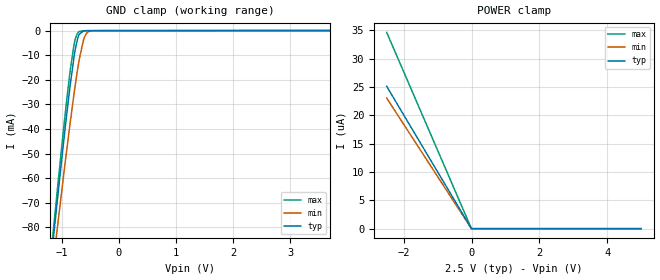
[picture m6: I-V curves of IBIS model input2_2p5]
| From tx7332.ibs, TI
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|   input2_2p5 Model
[Model]   input2_2p5
Model_type   Input
Vinl = 0.625
Vinh = 1.875
|   typ   min   max
C_comp   2.990pF   2.962pF   3.032pF
[Model spec]
|subparameter
Vinl   0.625   0.6   0.65
Vinh   1.875   1.8   1.95
| Where Nom  PVT is Nominal Process, 2.5V, 27C
|   Fast PVT is Strong Process,  2.6V, 0C
|   Slow PVT is Weak Process,   2.4V, 100C
[Voltage Range]   2.5   2.4   2.6
|Junction Temperature
[Temperature Range]   27   100   0
[Power Clamp Reference]   2.5   2.4   2.6
[GND Clamp Reference]   0   0   0
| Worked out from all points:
|   GND clamp passes 1 mA (typ) near -0.66 V on its own axis
[GND Clamp]
|   Voltage   I(typ)   I(min)   I(max)
-2.5V     -400.5mA   -375.1mA   -414.6mA
-1.173V   -90.47mA   -99.43mA   -87.36mA
-1.075V   -68.76mA   -80.04mA   -64.5mA
-955mV    -42.91mA   -56.73mA   -37.42mA
-850mV    -21.96mA   -37.2mA    -16.05mA
-767.5mV  -8.359mA   -22.95mA   -3.947mA
-722.5mV  -3.393mA   -15.91mA   -1.059mA
-692.5mV  -1.506mA   -11.69mA   -391.4uA
-595mV    -80.32uA   -2.351mA   -55.26uA
-542.5mV  -37.61uA   -643uA     -45.47uA
-467.5mV  -30.19uA   -97.15uA   -42.6uA
5V        0A         0A         0A
[POWER Clamp]
|   Voltage   I(typ)   I(min)   I(max)
-2.5V     25.1uA     23.03uA    34.61uA
-10mV     77nA       69.01nA    115nA
-2.5mV    1.652nA    34.51nA    11.22nA
5V        0A         0A         0A
